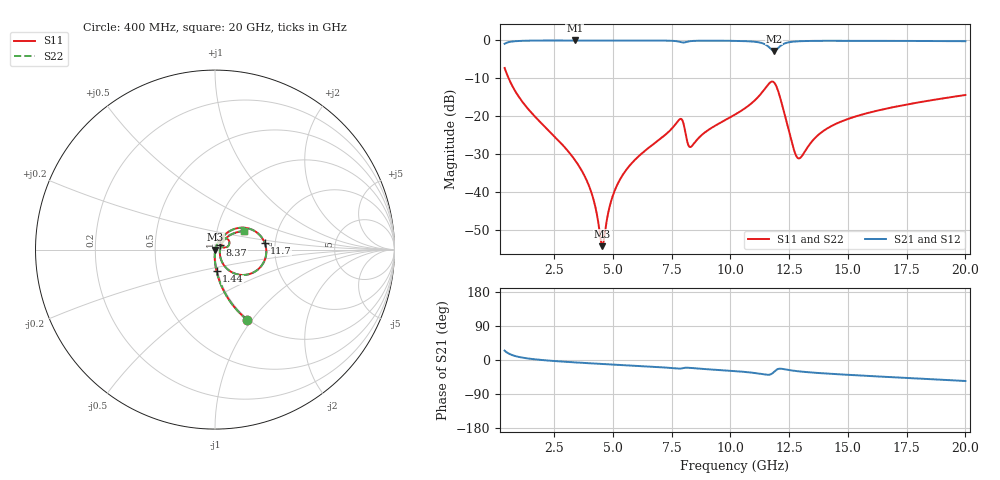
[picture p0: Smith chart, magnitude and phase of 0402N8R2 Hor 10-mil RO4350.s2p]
# MHz S  dB  R 50
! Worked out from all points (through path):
!   1961 points, 400 MHz to 20 GHz, reference 50 ohm
!   highest |S21| = -0.02 dB at 3.38 GHz (marker M1); lowest = -2.8 dB at 11.86 GHz (marker M2)
!   group delay of S21, straight-line fit = 8.42 ps
!   lowest |S11| = -54.3 dB at 4.56 GHz (marker M3), VSWR 1.00, Z = 50.2 - j0.0292 ohm
!   |S11| at or under -10 dB: 570.9 MHz to end of sweep
!   |S22| runs from -54.3 to -7.3 dB; largest |S21 - S12| = 0
!   S11 on the Smith chart (normalised r, x): 400 MHz: 0.99, -0.95; 1.44 GHz: 0.99, -0.24; 8.37 GHz: 1.06, +0.06; 11.7 GHz: 1.76, +0.15; 20 GHz: 1.34, +0.29
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400  -7.28 -65.2  -0.90 24.7  -0.90 24.7  -7.28 -65.2
1440  -18.37 -85.9  -0.07 3.6  -0.07 3.6  -18.37 -85.9
3380  -31.46 -92.8  -0.02 -6.3  -0.02 -6.3  -31.46 -92.8
3670  -34.24 -92.4  -0.02 -7.4  -0.02 -7.4  -34.24 -92.4
4150  -41.29 -86.9  -0.02 -9.1  -0.02 -9.1  -41.29 -86.9
4560  -54.28 -8.6  -0.02 -10.5  -0.02 -10.5  -54.28 -8.6
4920  -42.61 62.3  -0.02 -11.7  -0.02 -11.7  -42.61 62.3
5300  -36.78 68.3  -0.02 -13.0  -0.02 -13.0  -36.78 68.3
6940  -26.36 66.7  -0.05 -18.7  -0.05 -18.7  -26.36 66.7
7880  -20.70 37.3  -0.44 -22.7  -0.44 -22.7  -20.70 37.3
8220  -27.69 23.3  -0.27 -20.5  -0.27 -20.5  -27.69 23.3
8370  -27.83 43.8  -0.16 -21.3  -0.16 -21.3  -27.83 43.8
10200  -19.57 55.8  -0.13 -29.3  -0.13 -29.3  -19.57 55.8
11360  -13.66 35.8  -0.73 -37.3  -0.73 -37.3  -13.66 35.8
11700  -11.08 8.0  -2.10 -38.3  -2.10 -38.3  -11.08 8.0
11860  -11.09 -15.8  -2.76 -31.2  -2.76 -31.2  -11.09 -15.8
12260  -18.28 -58.4  -0.95 -23.9  -0.95 -23.9  -18.28 -58.4
12820  -30.64 -23.3  -0.26 -29.3  -0.26 -29.3  -30.64 -23.3
13470  -26.67 39.0  -0.14 -33.1  -0.14 -33.1  -26.67 39.0
14600  -21.71 46.6  -0.11 -37.7  -0.11 -37.7  -21.71 46.6
16740  -17.86 42.4  -0.13 -44.9  -0.13 -44.9  -17.86 42.4
20000  -14.41 33.0  -0.22 -55.4  -0.22 -55.4  -14.41 33.0
